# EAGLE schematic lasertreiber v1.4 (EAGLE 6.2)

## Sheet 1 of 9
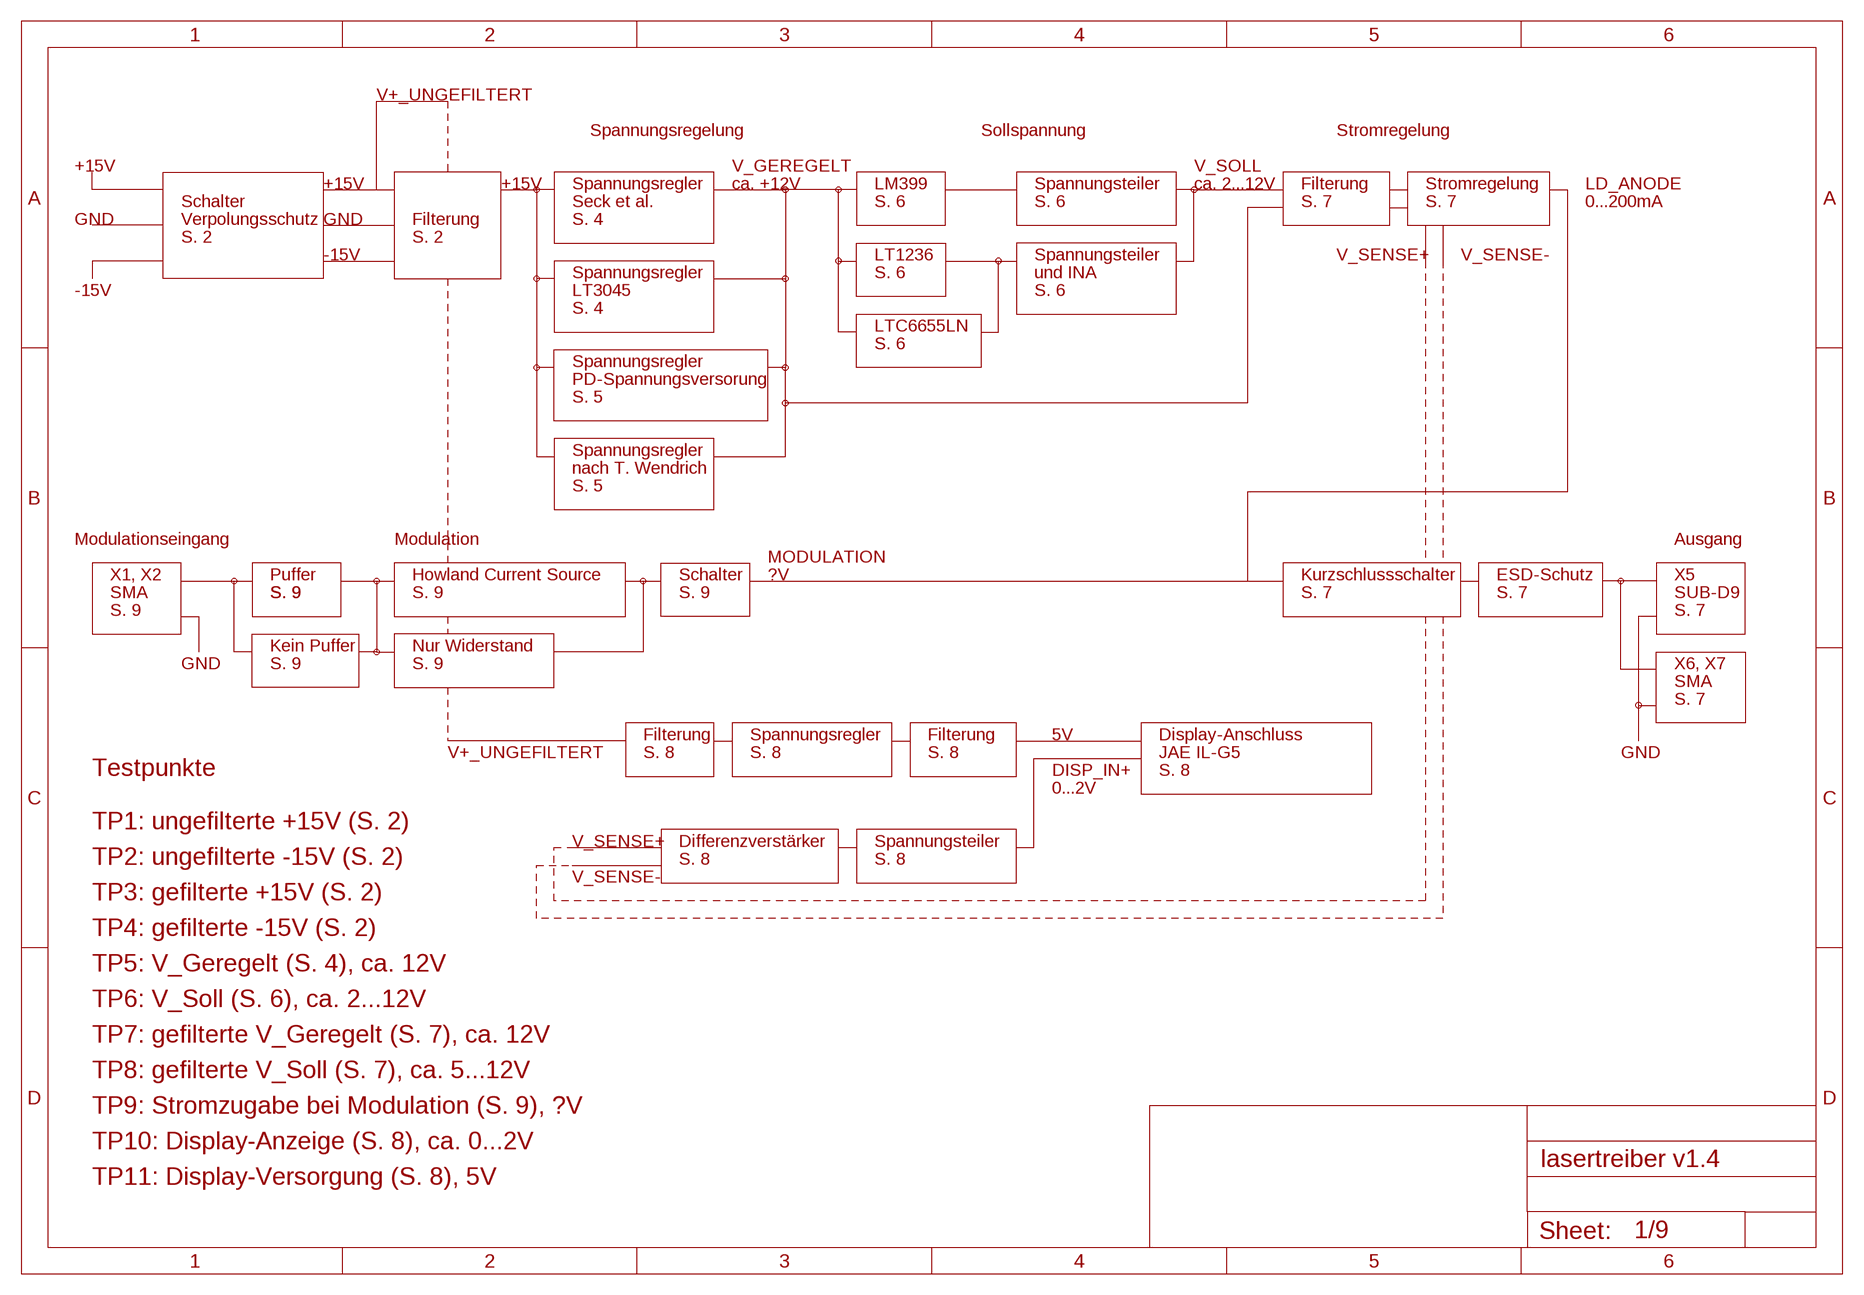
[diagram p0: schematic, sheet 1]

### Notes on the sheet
- V+_UNGEFILTERT
- Spannungsregelung | Sollspannung | Stromregelung
- +15V | V_GEREGELT | V_SOLL
- +15V | +15V | Spannungsregler | ca. +12V | LM399 | Spannungsteiler | ca. 2...12V | Filterung | Stromregelung | LD_ANODE
- Schalter | Seck et al. | S. 6 | S. 6 | S. 7 | S. 7 | 0...200mA
- GND | Verpolungsschutz | GND | Filterung | S. 4
- S. 2 | S. 2
- -15V | LT1236 | Spannungsteiler | V_SENSE+ | V_SENSE-
- Spannungsregler | S. 6 | und INA
- -15V | LT3045 | S. 6
- S. 4
- LTC6655LN
- S. 6
- Spannungsregler
- PD-Spannungsversorung
- S. 5
- Spannungsregler
- nach T. Wendrich
- S. 5
- Modulationseingang | Modulation | Ausgang
- MODULATION
- X1, X2 | Puffer | Howland Current Source | Schalter | ?V | Kurzschlussschalter | ESD-Schutz | X5
- SMA | S. 9 | S. 9 | S. 9 | S. 9 | S. 7 | S. 7 | SUB-D9
- S. 9 | S. 7
- Kein Puffer | Nur Widerstand
- GND | S. 9 | S. 9 | X6, X7
- SMA
- S. 7
- Filterung | Spannungsregler | Filterung | 5V | Display-Anschluss
- V+_UNGEFILTERT | S. 8 | S. 8 | S. 8 | JAE IL-G5 | GND
- Testpunkte | DISP_IN+ | S. 8
- 0...2V
- TP1: ungefilterte +15V (S. 2)
- V_SENSE+ | Differenzverstärker | Spannungsteiler
- TP2: ungefilterte -15V (S. 2) | S. 8 | S. 8
- V_SENSE-
- TP3: gefilterte +15V (S. 2)
- TP4: gefilterte -15V (S. 2)
- TP5: V_Geregelt (S. 4), ca. 12V
- TP6: V_Soll (S. 6), ca. 2...12V
- TP7: gefilterte V_Geregelt (S. 7), ca. 12V
- TP8: gefilterte V_Soll (S. 7), ca. 5...12V
- TP9: Stromzugabe bei Modulation (S. 9), ?V
- TP10: Display-Anzeige (S. 8), ca. 0...2V
- TP11: Display-Versorgung (S. 8), 5V

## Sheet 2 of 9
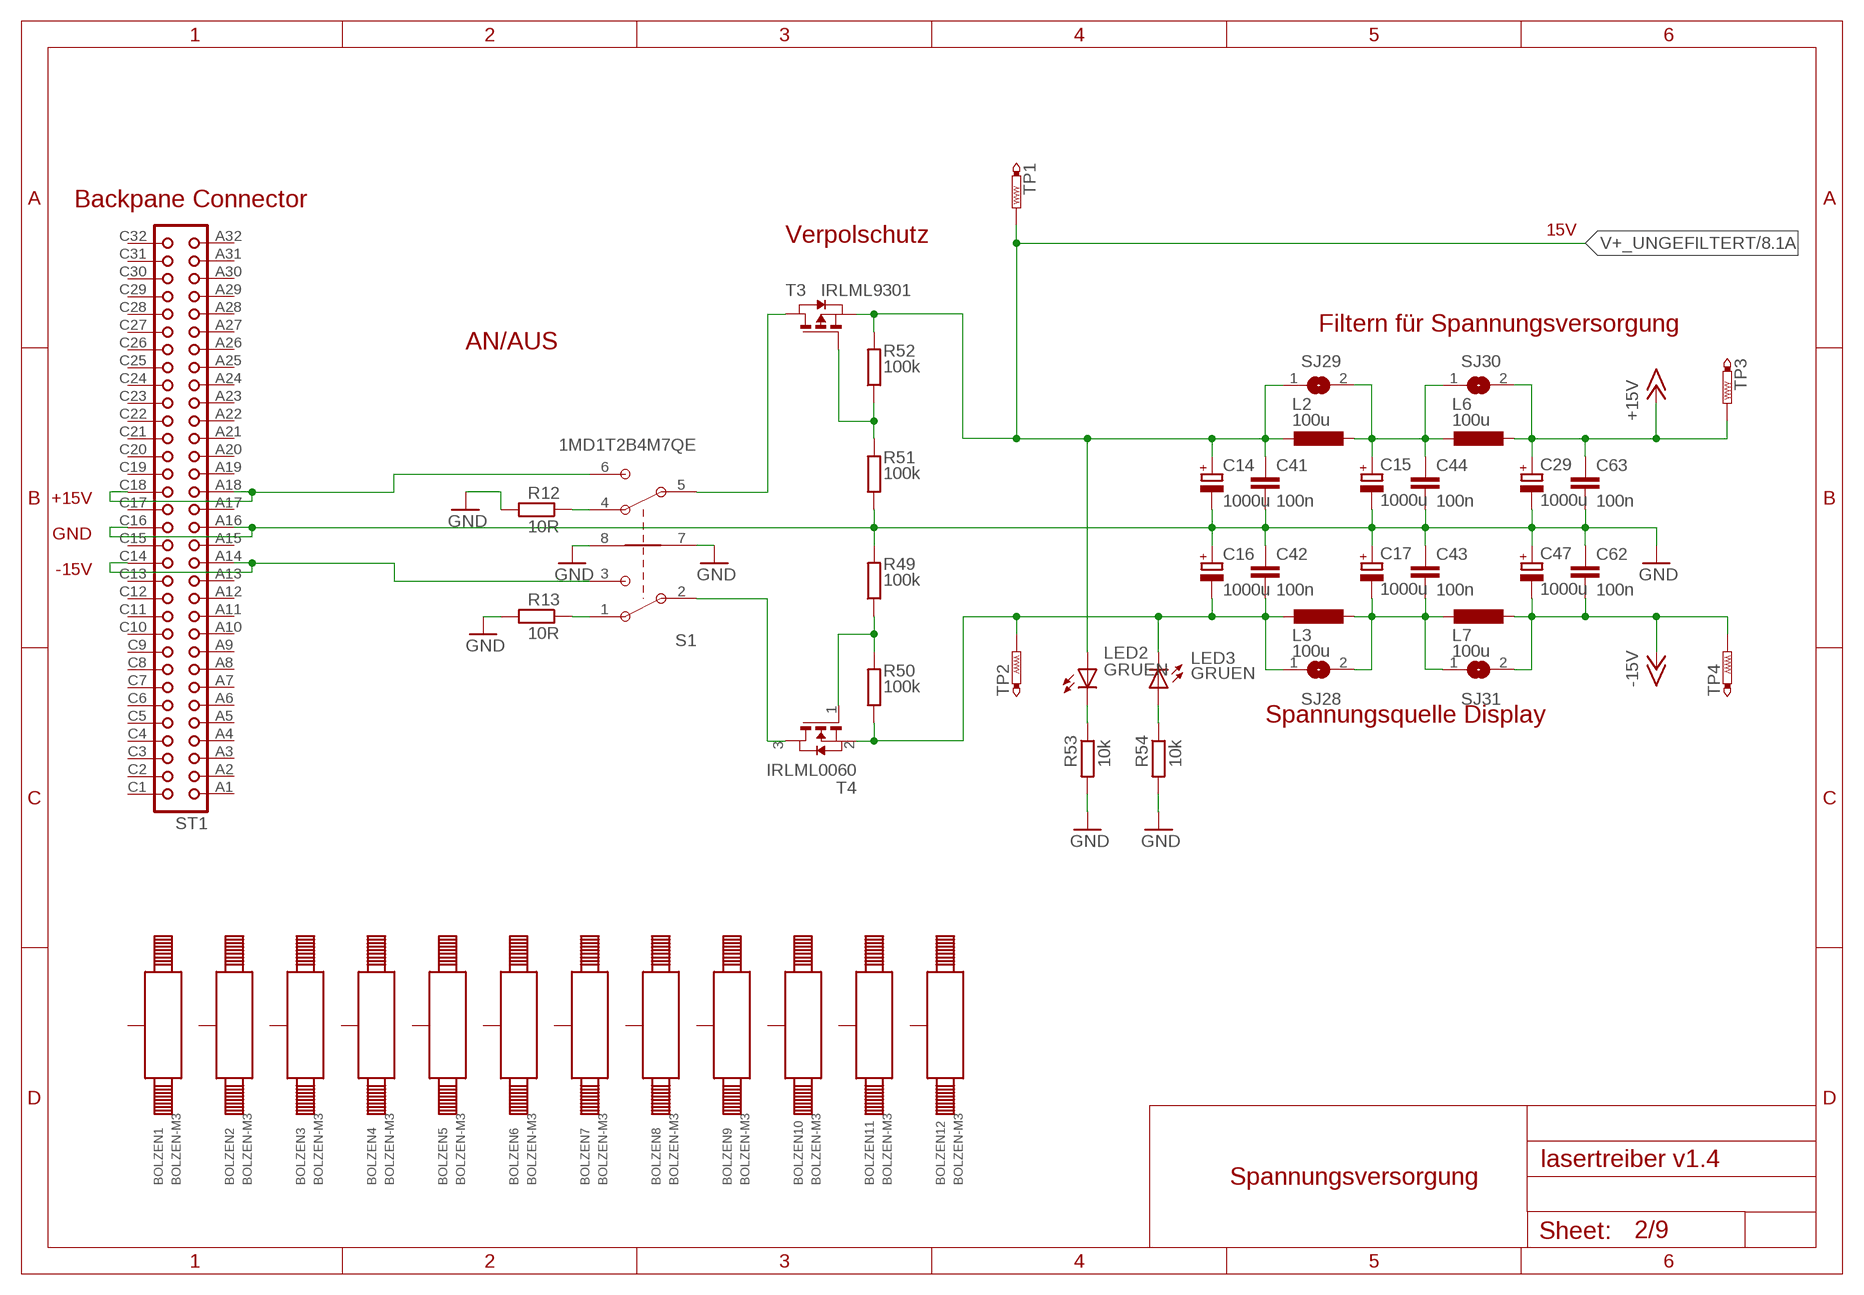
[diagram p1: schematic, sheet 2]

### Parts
BOLZEN1  BOLZEN-M3  [LOCH-M3]
BOLZEN2  BOLZEN-M3  [LOCH-M3]
BOLZEN3  BOLZEN-M3  [LOCH-M3]
BOLZEN4  BOLZEN-M3  [LOCH-M3]
BOLZEN5  BOLZEN-M3  [LOCH-M3]
BOLZEN6  BOLZEN-M3  [LOCH-M3]
BOLZEN7  BOLZEN-M3  [LOCH-M3]
BOLZEN8  BOLZEN-M3  [LOCH-M3]
BOLZEN9  BOLZEN-M3  [LOCH-M3]
BOLZEN10  BOLZEN-M3  [LOCH-M3]
BOLZEN11  BOLZEN-M3  [LOCH-M3]
BOLZEN12  BOLZEN-M3  [LOCH-M3]
C14  1000u  C-POL1000UF  [TT5D10]
C15  1000u  C-POL1000UF  [TT5D10]
C16  1000u  C-POL1000UF  [TT5D10]
C17  1000u  C-POL1000UF  [TT5D10]
C29  1000u  C-POL1000UF  [TT5D10]
C41  100n  C0805  [C0805]
C42  100n  C0805  [C0805]
C43  100n  C0805  [C0805]
C44  100n  C0805  [C0805]
C47  1000u  C-POL1000UF  [TT5D10]
C62  100n  C0805  [C0805]
C63  100n  C0805  [C0805]
L2  100u  L2100MA100UH  [L-GROSS]
L3  100u  L2100MA100UH  [L-GROSS]
L6  100u  L2100MA100UH  [L-GROSS]
L7  100u  L2100MA100UH  [L-GROSS]
LED2  GRUEN  LED3MM-GRUEN  [LED3MM]
LED3  GRUEN  LED3MM-GRUEN  [LED3MM]
R12  10R  R0805  [R0805]
R13  10R  R0805  [R0805]
R49  100k  R0805  [R0805]
R50  100k  R0805  [R0805]
R51  100k  R0805  [R0805]
R52  100k  R0805  [R0805]
R53  10k  R0805  [R0805]
R54  10k  R0805  [R0805]
S1  1MD1T2B4M7QE  [1MD1T2B4M7QE]
SJ28  SJ  [SJ]
SJ29  SJ  [SJ]
SJ30  SJ  [SJ]
SJ31  SJ  [SJ]
ST1  A.KO-09_MAC64LEMESSERLEISTE  [A.KO-09_MAC64L]
T3  IRLML9301  [SOT23]
T4  IRLML0060  [SOT23]
TP1  PTR1PAD1-13  [P1-13]
TP2  PTR1PAD1-13  [P1-13]
TP3  PTR1PAD1-13  [P1-13]
TP4  PTR1PAD1-13  [P1-13]

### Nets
+15V: C29.+ C63.1 L6.P$2 SJ30.2 TP3.TP ; also sheet 3,4,5,6,7,8
-15V: C47.- C62.2 L7.P$2 SJ31.2 TP4.TP ; also sheet 3,6,7,8
GND: C14.- C15.- C16.+ C17.+ C29.- C41.2 C42.1 C43.1 C44.2 C47.+ C62.1 C63.2 R12.2 R13.2 R49.2 R51.1 R53.2 R54.2 S1.7(GND) S1.8(GND) ST1.A16 ST1.C16 ; also sheet 3,4,5,6,7,8,9
N$16: C15.+ C44.1 L2.P$2 L6.P$1 SJ29.2 SJ30.1
N$17: R12.1 S1.4(B1)
N$18: R13.1 S1.1(A1)
N$40: S1.2(A) T4.3(D)
N$54: LED3.A R54.1
N$73: S1.6(B2) ST1.A18 ST1.C18
N$86: R51.2 R52.1 T3.1(G)
N$89: R49.1 R50.2 T4.1(G)
N$97: S1.5(B) T3.3(D)
N$162: S1.3(A2) ST1.A14 ST1.C14
N$175: LED2.K(C) R53.1
V+_UNGEFILTERT: C14.+ C41.1 L2.P$1 LED2.A R52.2 SJ29.1 T3.2(S) TP1.TP ; also sheet 8
V-: C17.- C43.2 L3.P$2 L7.P$1 SJ28.2 SJ31.1
V-_UNGEFILTERT: C16.- C42.2 L3.P$1 LED3.K(C) R50.1 SJ28.1 T4.2(S) TP2.TP
Unconnected: BOLZEN1.1 BOLZEN2.1 BOLZEN3.1 BOLZEN4.1 BOLZEN5.1 BOLZEN6.1 BOLZEN7.1 BOLZEN8.1 BOLZEN9.1 BOLZEN10.1 BOLZEN11.1 BOLZEN12.1 ST1.A1 ST1.A2 ST1.A3 ST1.A4 ST1.A5 ST1.A6 ST1.A7 ST1.A8 ST1.A9 ST1.A10 ST1.A11 ST1.A12 ST1.A13 ST1.A15 ST1.A17 ST1.A19 ST1.A20 ST1.A21 ST1.A22 ST1.A23 ST1.A24 ST1.A25 ST1.A26 ST1.A27 ST1.A28 ST1.A29 ST1.A30 ST1.A31 ST1.A32 ST1.C1 ST1.C2 ST1.C3 ST1.C4 ST1.C5 ST1.C6 ST1.C7 ST1.C8 ST1.C9 ST1.C10 ST1.C11 ST1.C12 ST1.C13 ST1.C15 ST1.C17 ST1.C19 ST1.C20 ST1.C21 ST1.C22 ST1.C23 ST1.C24 ST1.C25 ST1.C26 ST1.C27 ST1.C28 ST1.C29 ST1.C30 ST1.C31 ST1.C32

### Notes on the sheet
- Backpane Connector
- 15V
- Verpolschutz
- Filtern für Spannungsversorgung
- AN/AUS
- +15V
- GND
- -15V
- Spannungsquelle Display
- Spannungsversorgung

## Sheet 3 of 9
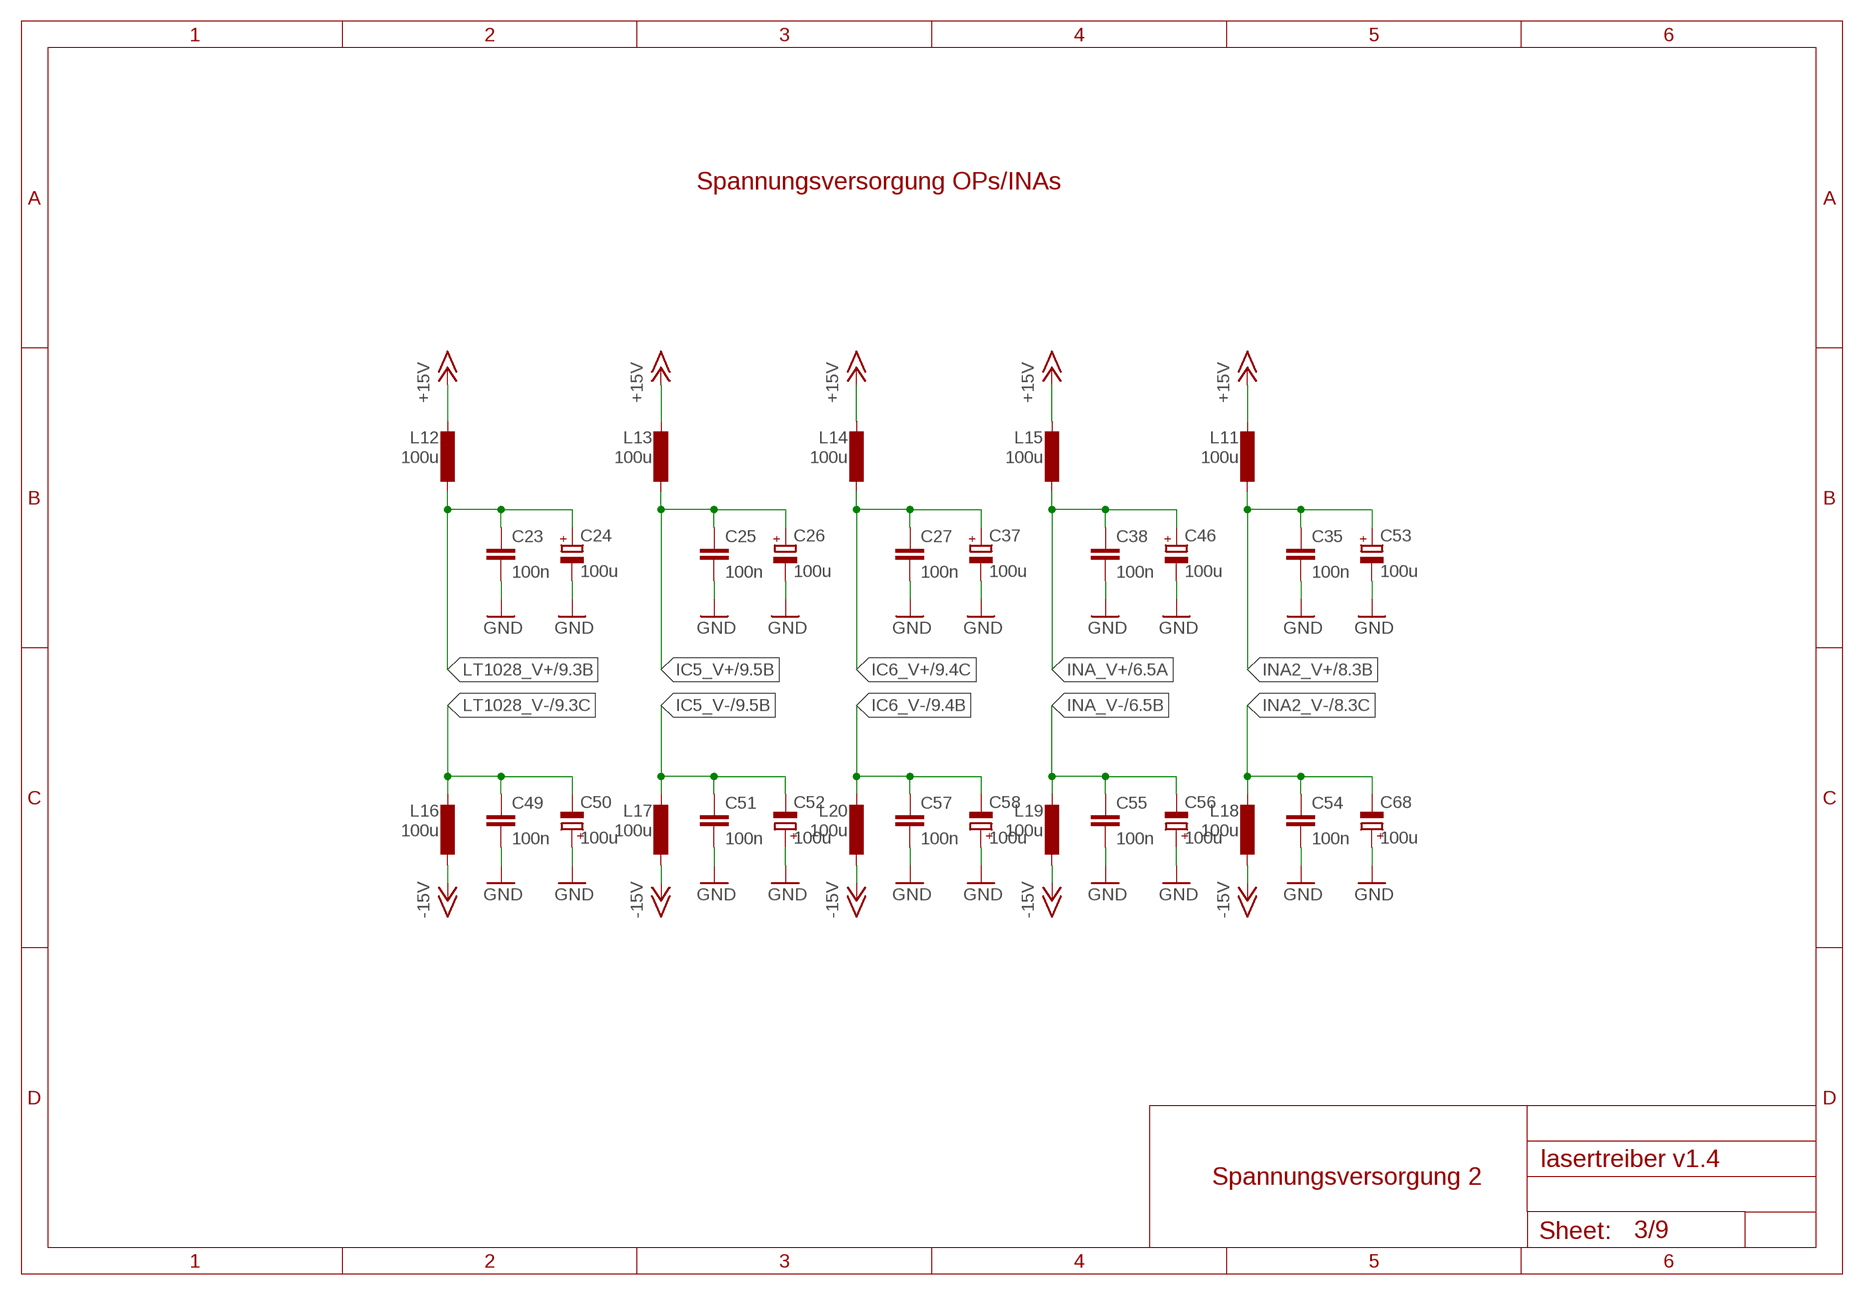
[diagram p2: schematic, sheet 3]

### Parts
C23  100n  C0805  [C0805]
C24  100u  C-POL100UF  [TT5D7]
C25  100n  C0805  [C0805]
C26  100u  C-POL100UF  [TT5D7]
C27  100n  C0805  [C0805]
C35  100n  C0805  [C0805]
C37  100u  C-POL100UF  [TT5D7]
C38  100n  C0805  [C0805]
C46  100u  C-POL100UF  [TT5D7]
C49  100n  C0805  [C0805]
C50  100u  C-POL100UF  [TT5D7]
C51  100n  C0805  [C0805]
C52  100u  C-POL100UF  [TT5D7]
C53  100u  C-POL100UF  [TT5D7]
C54  100n  C0805  [C0805]
C55  100n  C0805  [C0805]
C56  100u  C-POL100UF  [TT5D7]
C57  100n  C0805  [C0805]
C58  100u  C-POL100UF  [TT5D7]
C68  100u  C-POL100UF  [TT5D7]
L11  100u  L100MA100UH  [L-KLEIN]
L12  100u  L100MA100UH  [L-KLEIN]
L13  100u  L100MA100UH  [L-KLEIN]
L14  100u  L100MA100UH  [L-KLEIN]
L15  100u  L100MA100UH  [L-KLEIN]
L16  100u  L100MA100UH  [L-KLEIN]
L17  100u  L100MA100UH  [L-KLEIN]
L18  100u  L100MA100UH  [L-KLEIN]
L19  100u  L100MA100UH  [L-KLEIN]
L20  100u  L100MA100UH  [L-KLEIN]

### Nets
+15V: L11.2 L12.2 L13.2 L14.2 L15.2 ; also sheet 2,4,5,6,7,8
-15V: L16.1 L17.1 L18.1 L19.1 L20.1 ; also sheet 2,6,7,8
GND: C23.2 C24.- C25.2 C26.- C27.2 C35.2 C37.- C38.2 C46.- C49.2 C50.+ C51.2 C52.+ C53.- C54.2 C55.2 C56.+ C57.2 C58.+ C68.+ ; also sheet 2,4,5,6,7,8,9
IC5_V+: C25.1 C26.+ L13.1 ; also sheet 9
IC5_V-: C51.1 C52.- L17.2 ; also sheet 9
IC6_V+: C27.1 C37.+ L14.1 ; also sheet 9
IC6_V-: C57.1 C58.- L20.2 ; also sheet 9
INA2_V+: C35.1 C53.+ L11.1 ; also sheet 8
INA2_V-: C54.1 C68.- L18.2 ; also sheet 8
INA_V+: C38.1 C46.+ L15.1 ; also sheet 6
INA_V-: C55.1 C56.- L19.2 ; also sheet 6
LT1028_V+: C23.1 C24.+ L12.1 ; also sheet 9
LT1028_V-: C49.1 C50.- L16.2 ; also sheet 9

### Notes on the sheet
- Spannungsversorgung OPs/INAs
- Spannungsversorgung 2

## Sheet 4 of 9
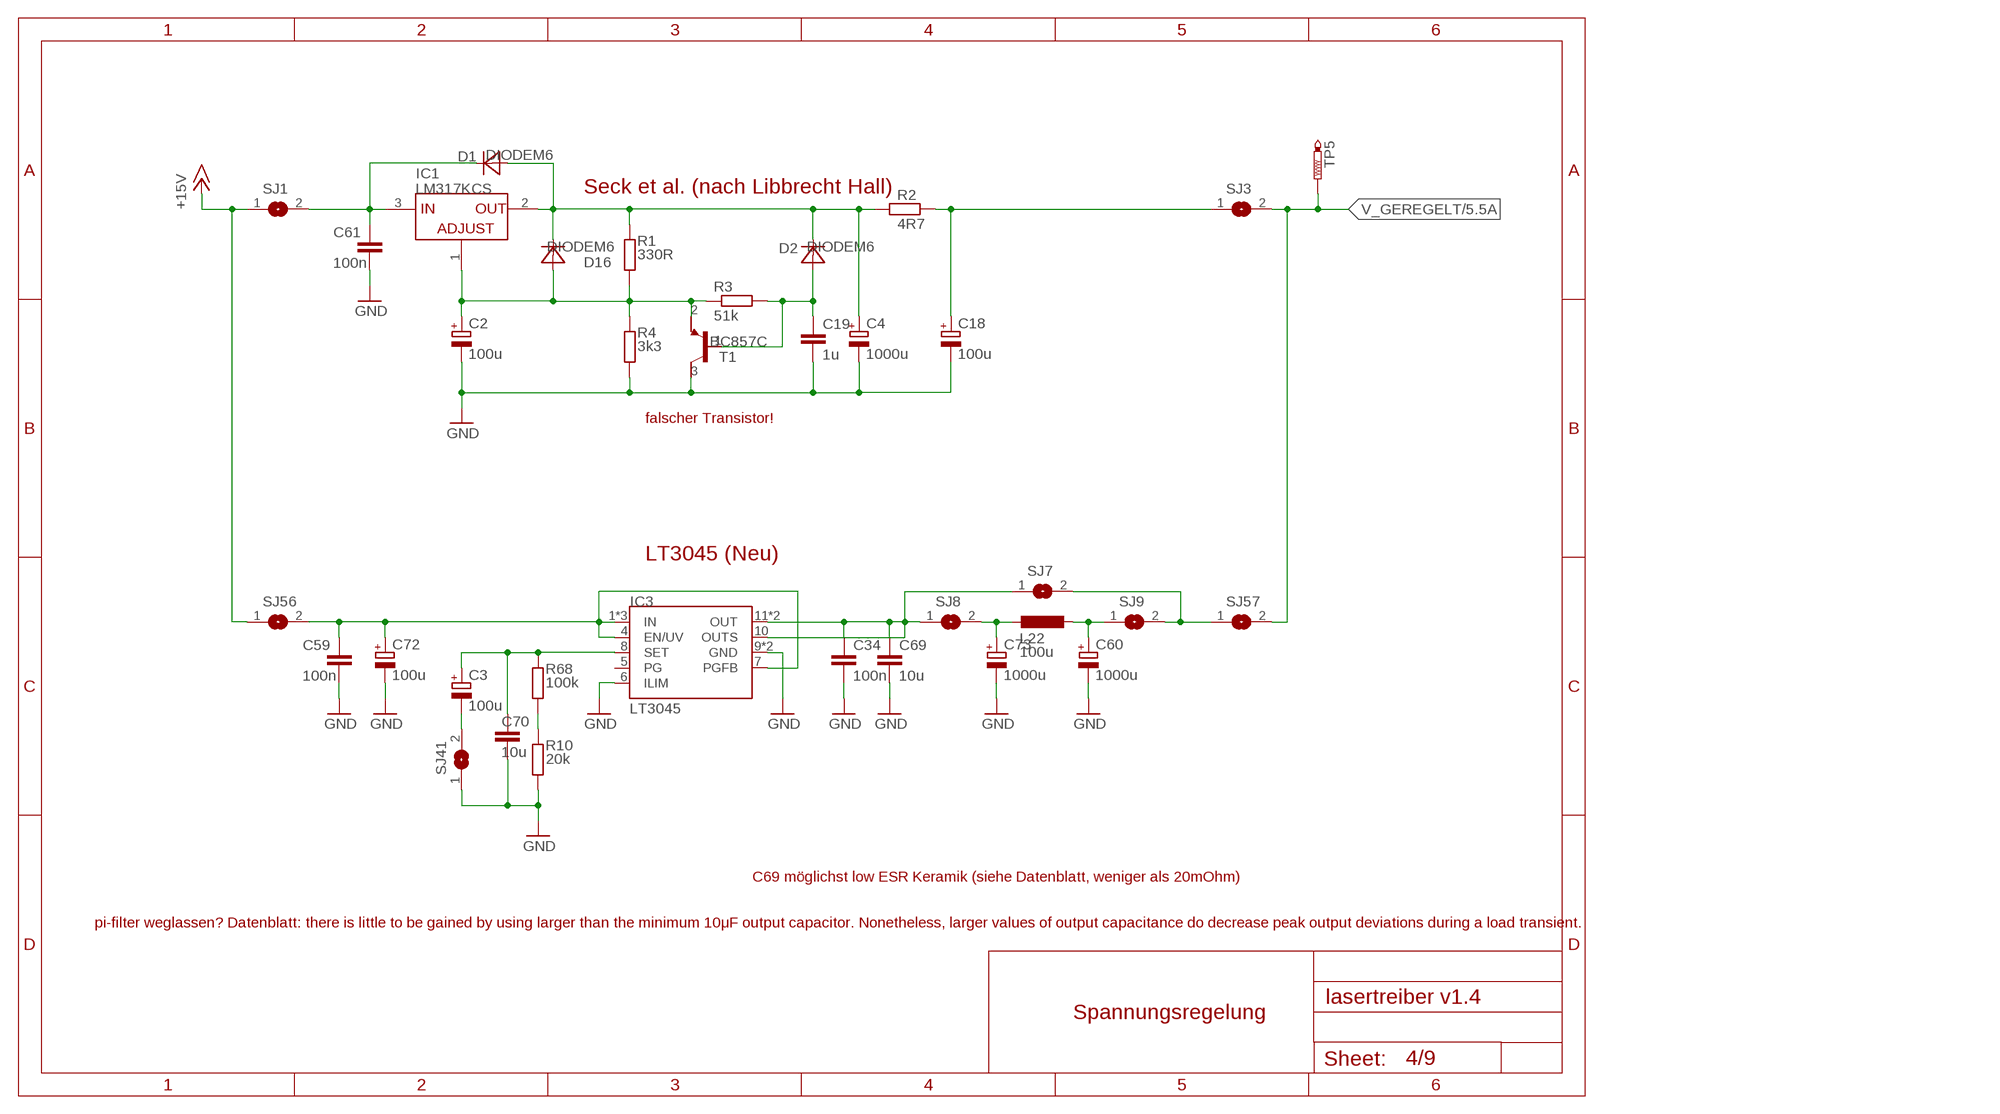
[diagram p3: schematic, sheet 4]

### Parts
C2  100u  C-POL100UF  [TT5D7]
C3  100u  C-POL100UF  [TT5D7]
C4  1000u  C-POL1000UF  [TT5D10]
C18  100u  C-POL100UF  [TT5D7]
C19  1u  C50X75  [C050-050X075]
C34  100n  C0805  [C0805]
C59  100n  C0805  [C0805]
C60  1000u  C-POL1000UF  [TT5D10]
C61  100n  C0805  [C0805]
C69  10u  CMKS2B051001N00KSSD  [MKS2]
C70  10u  CMKS2B051001N00KSSD  [MKS2]
C72  100u  C-POL100UF  [TT5D7]
C73  1000u  C-POL1000UF  [TT5D10]
D1  DIODEM6  [DIODE]
D2  DIODEM6  [DIODE]
D16  DIODEM6  [DIODE]
IC1  LM317KCS  [TO220]
IC3  LT3045  [MSE]
L22  100u  L2100MA100UH  [L-GROSS]
R1  330R  R0805  [R0805]
R2  4R7  R1206  [R1206]
R3  51k  R0805  [R0805]
R4  3k3  R0805  [R0805]
R10  20k  R0805  [R0805]
R68  100k  R0805  [R0805]
SJ1  SJ  [SJ]
SJ3  SJ  [SJ]
SJ7  SJ  [SJ]
SJ8  SJ  [SJ]
SJ9  SJ  [SJ]
SJ41  SJ  [SJ]
SJ56  SJ  [SJ]
SJ57  SJ  [SJ]
T1  BC857C  [SOT23]
TP5  PTR1PAD1-13  [P1-13]

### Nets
+15V: SJ1.1 SJ56.1 ; also sheet 2,3,5,6,7,8
GND: C2.- C4.- C18.- C19.1 C34.1 C59.1 C60.- C61.1 C69.1 C70.1 C72.- C73.- IC3.6(ILIM) IC3.9(GND) IC3.13(GND) R4.1 R10.1 SJ41.1 T1.3(C) ; also sheet 2,3,5,6,7,8,9
N$2: C19.2 D2.ANODE(A) R3.2 T1.1(B)
N$3: C2.+ D16.ANODE(A) IC1.1(ADJUST) R1.1 R3.1 R4.2 T1.2(E)
N$5: C4.+ D1.ANODE(A) D2.KATHODE(C) D16.KATHODE(C) IC1.2(OUT) R1.2 R2.2
N$9: R10.2 R68.1
N$33: C18.+ R2.1 SJ3.1
N$45: C34.2 C69.2 IC3.10(OUTS) IC3.11(OUT) IC3.12(OUT) SJ7.1 SJ8.1
N$46: C73.+ L22.P$1 SJ8.2
N$50: SJ7.2 SJ9.2 SJ57.1
N$51: C3.- SJ41.2
N$138: C3.+ C70.2 IC3.8(SET) R68.2
N$139: C59.2 C72.+ IC3.1(IN) IC3.2(IN) IC3.3(IN) IC3.4(EN/UV) IC3.7(PGFB) SJ56.2
N$142: C60.+ L22.P$2 SJ9.1
V+: C61.2 D1.KATHODE(C) IC1.3(INPUT) SJ1.2
V_GEREGELT: SJ3.2 SJ57.2 TP5.TP ; also sheet 5,6,7
Unconnected: IC3.5(PG)

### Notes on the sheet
- Seck et al. (nach Libbrecht Hall)
- falscher Transistor!
- LT3045 (Neu)
- C69 möglichst low ESR Keramik (siehe Datenblatt, weniger als 20mOhm)
- pi-filter weglassen? Datenblatt: there is little to be gained by using larger than the minimum 10μF output capacitor. Nonetheless, larger values of output capacitance do decrease peak output deviations during a load transient.
- Spannungsregelung

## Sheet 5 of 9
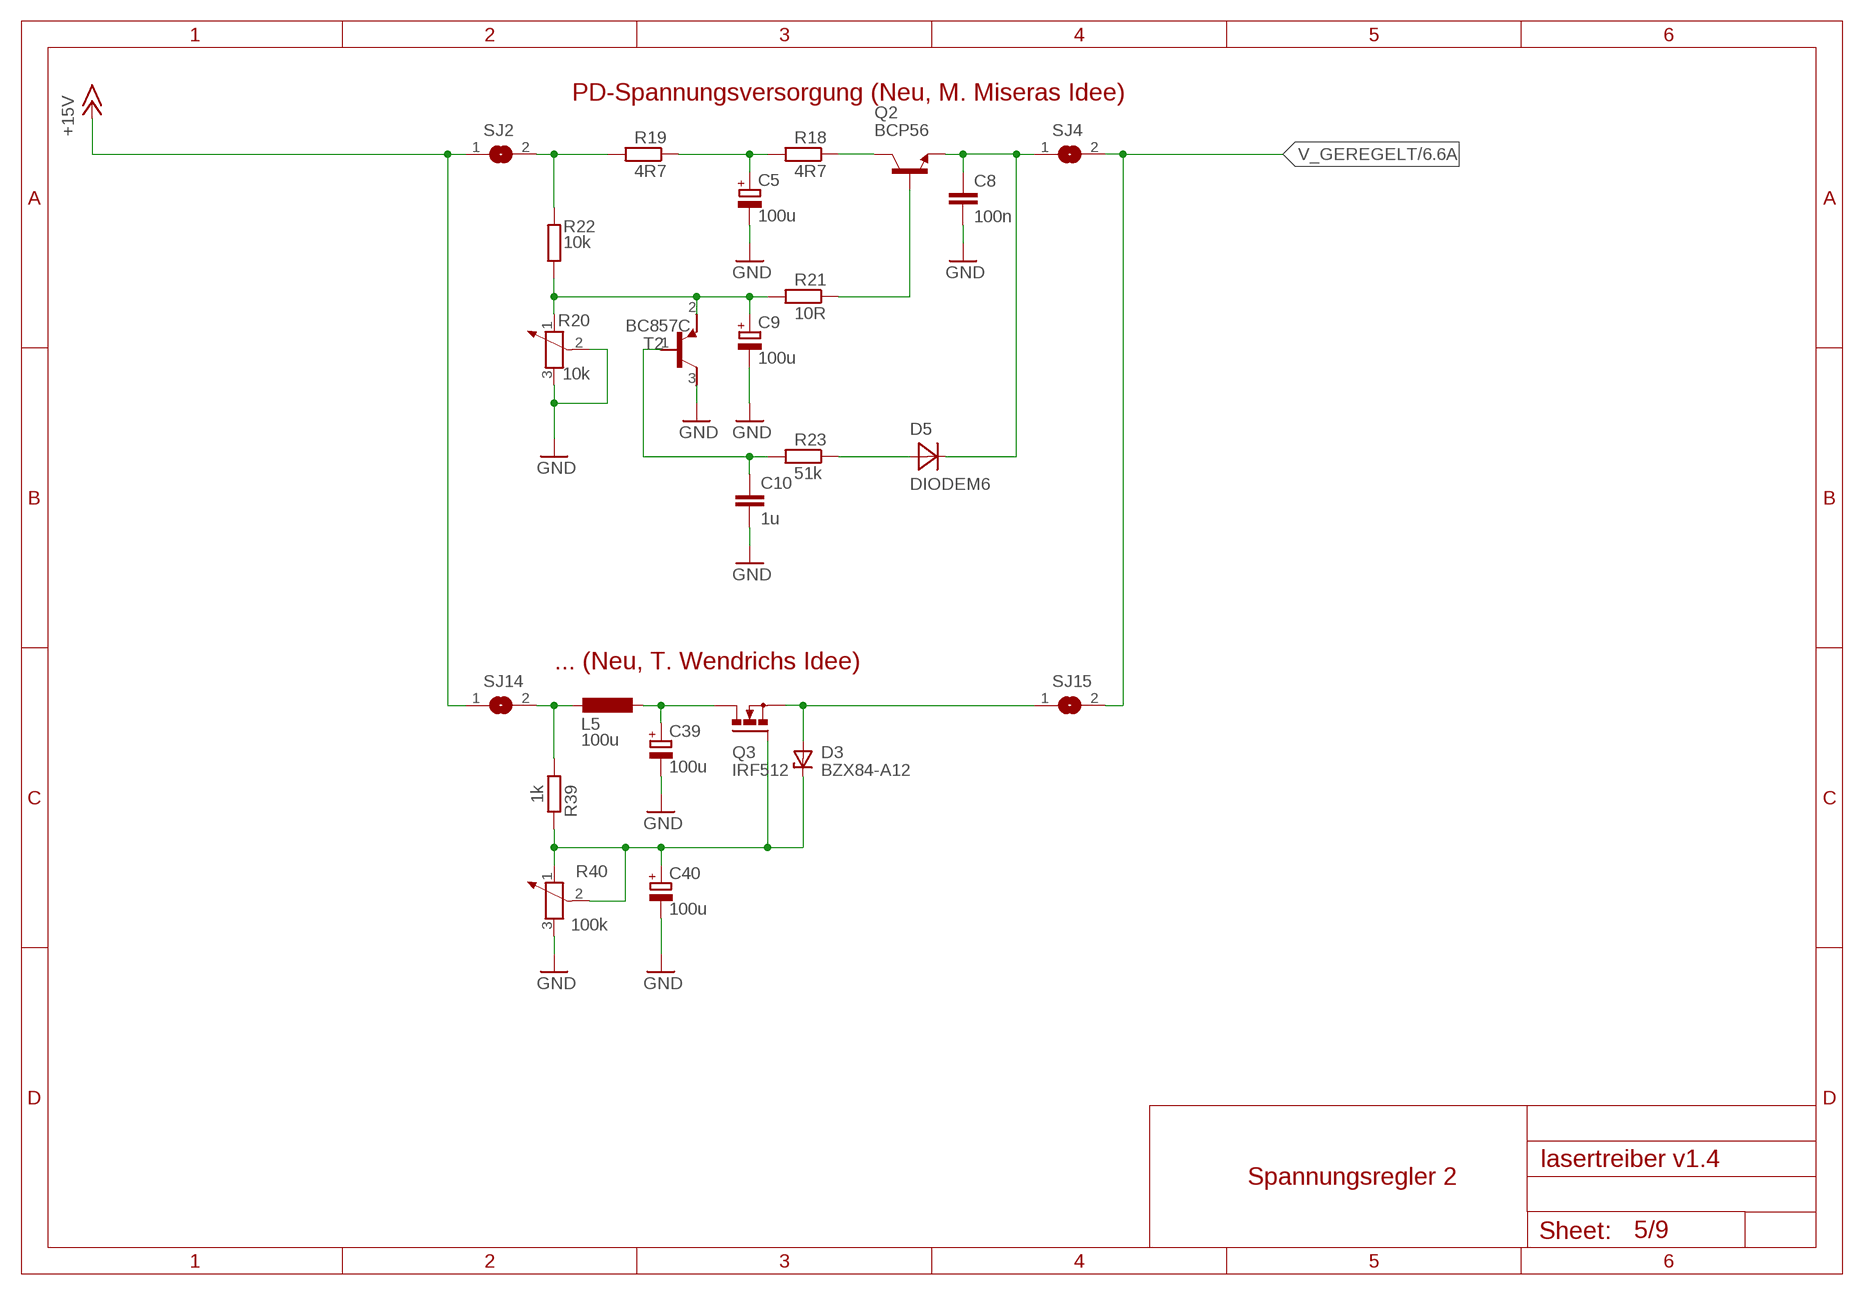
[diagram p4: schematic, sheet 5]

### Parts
C5  100u  C-POL100UF  [TT5D7]
C8  100n  C0805  [C0805]
C9  100u  C-POL100UF  [TT5D7]
C10  1u  C50X75  [C050-050X075]
C39  100u  C-POL100UF  [TT5D7]
C40  100u  C-POL100UF  [TT5D7]
D3  BZX84-A12  BZX84  [SOT23]
D5  DIODEM6  [DIODE]
L5  100u  L2100MA100UH  [L-GROSS]
Q2  BCP56  [SOT223]
Q3  IRF512  [TO220]
R18  4R7  R1206  [R1206]
R19  4R7  R1206  [R1206]
R20  10k  POTENTIOMETER_64Y  [64Y-POTI]
R21  10R  R0805  [R0805]
R22  10k  R0805  [R0805]
R23  51k  R0805  [R0805]
R39  1k  R0805  [R0805]
R40  100k  POTENTIOMETER_64Y  [64Y-POTI]
SJ2  SJ  [SJ]
SJ4  SJ  [SJ]
SJ14  SJ  [SJ]
SJ15  SJ  [SJ]
T2  BC857C  [SOT23]

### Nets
+15V: SJ2.1 SJ14.1 ; also sheet 2,3,4,6,7,8
GND: C5.- C8.1 C9.- C10.1 C39.- C40.- R20.2 R20.3 R40.3 T2.3(C) ; also sheet 2,3,4,6,7,8,9
N$24: C5.+ R18.2 R19.1
N$25: C8.2 D5.KATHODE(C) Q2.3(E) SJ4.1
N$26: Q2.2(C) Q2.4(C) R18.1
N$27: C9.+ R20.1 R21.2 R22.1 T2.2(E)
N$28: Q2.1(B) R21.1
N$29: C10.2 R23.2 T2.1(B)
N$30: R19.2 R22.2 SJ2.2
N$31: D5.ANODE(A) R23.1
N$32: C40.+ D3.3(K) Q3.1(G) R39.1 R40.1 R40.2
N$59: C39.+ L5.P$2 Q3.2(D)
N$60: L5.P$1 R39.2 SJ14.2
N$61: D3.1(A) Q3.3(S) SJ15.1
V_GEREGELT: SJ4.2 SJ15.2 ; also sheet 4,6,7

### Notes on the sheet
- PD-Spannungsversorgung (Neu, M. Miseras Idee)
- ... (Neu, T. Wendrichs Idee)
- Spannungsregler 2

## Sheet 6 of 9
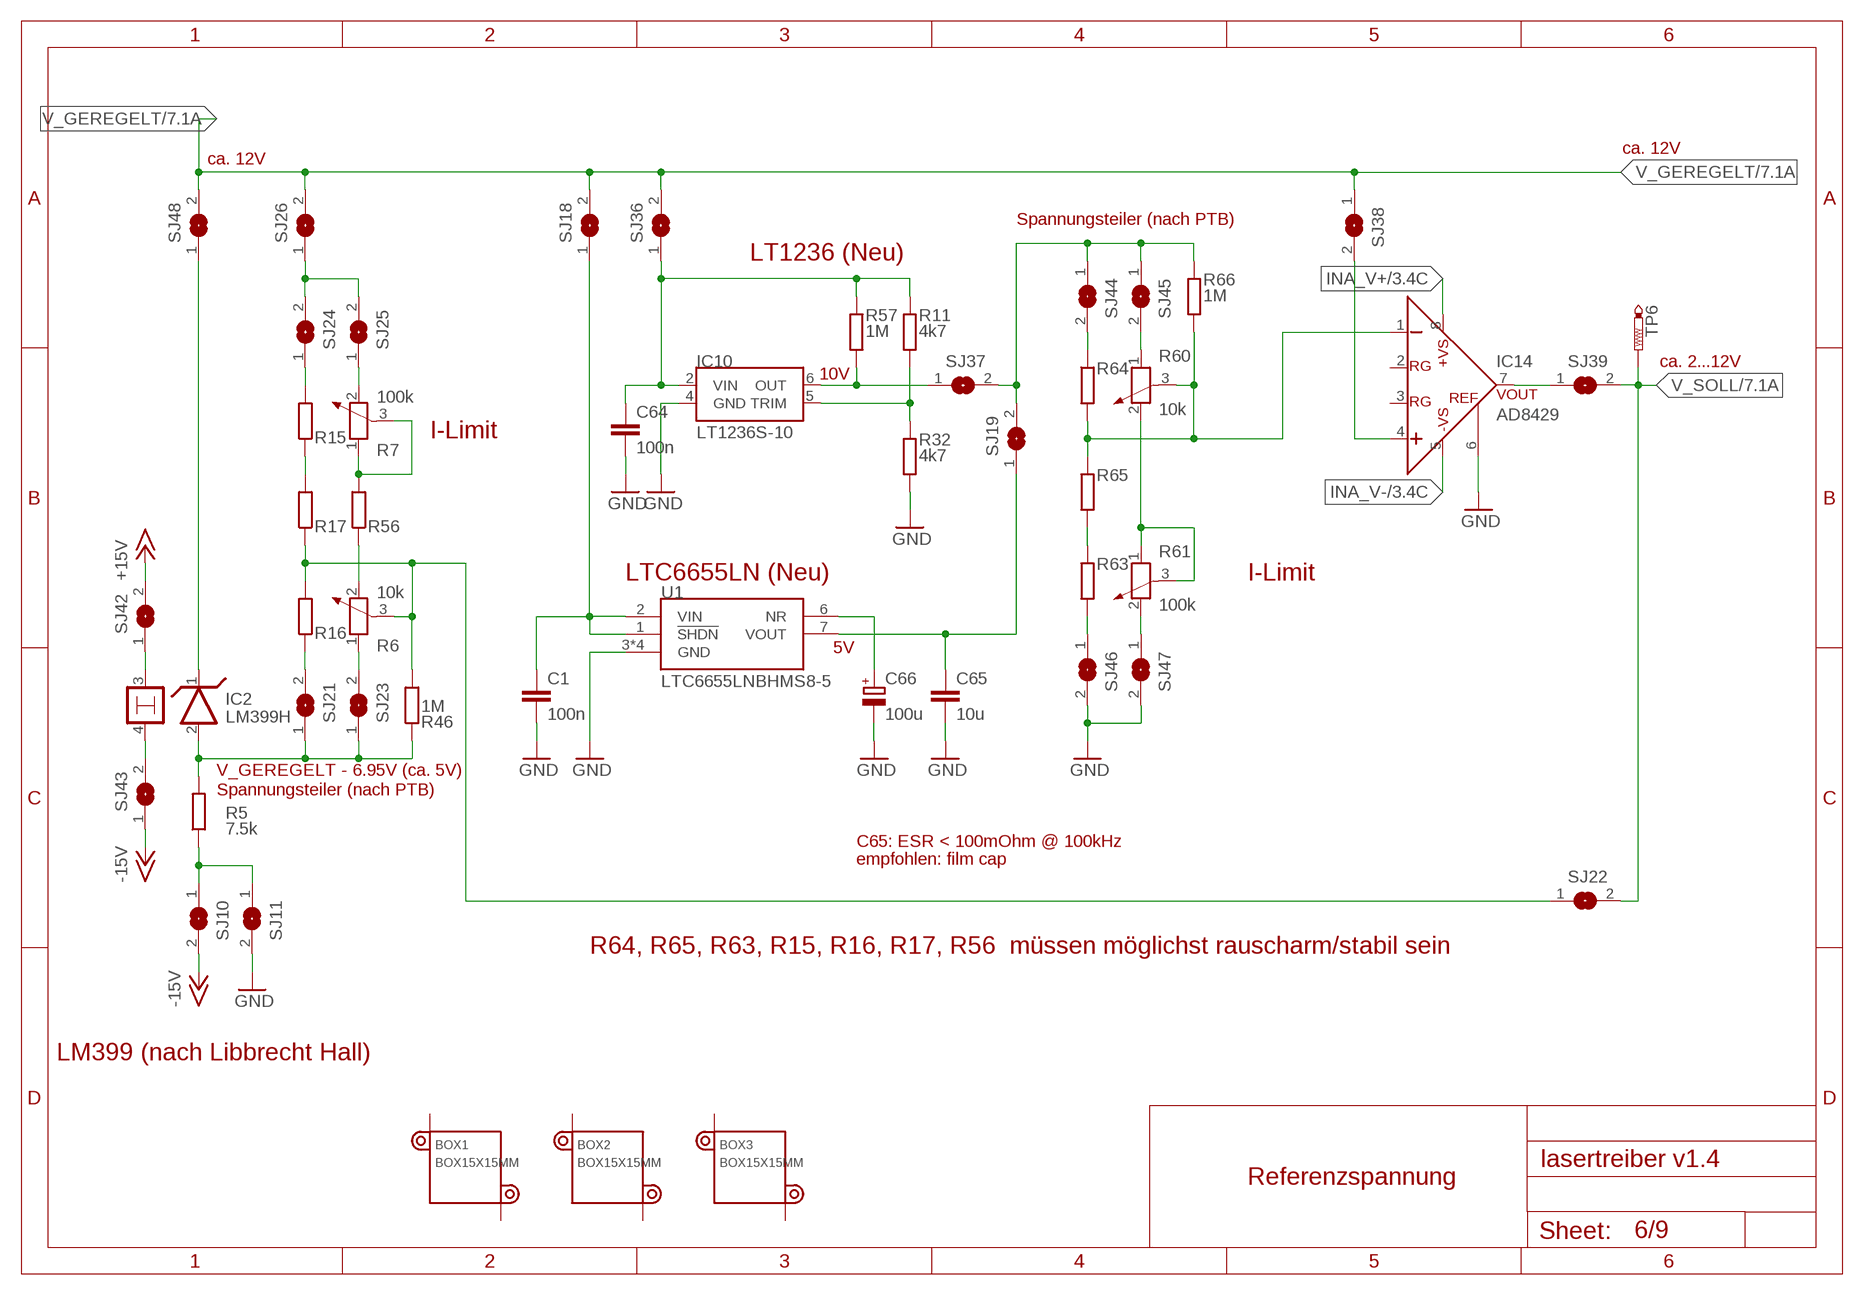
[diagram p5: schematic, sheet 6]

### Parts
BOX1  BOX15X15MM  [BOX-15X15MM]
BOX2  BOX15X15MM  [BOX-15X15MM]
BOX3  BOX15X15MM  [BOX-15X15MM]
C1  100n  C0805  [C0805]
C64  100n  C0805  [C0805]
C65  10u  CMKS2B051001N00KSSD  [MKS2]
C66  100u  C-POL100UF  [TT5D7]
IC2  LM399H  [TO39/4]
IC10  LT1236S-10  [SOIC8]
IC14  AD8429  [R-8]
R5  7.5k  R0805  [R0805]
R6  10k  POTENTIOMETER_PT-10  [PT-10]
R7  100k  POTENTIOMETER_PT-10  [PT-10]
R11  4k7  R0805  [R0805]
R15  R0805  [R0805]
R16  R0805  [R0805]
R17  R0805  [R0805]
R32  4k7  R0805  [R0805]
R46  1M  R0805  [R0805]
R56  R0805  [R0805]
R57  1M  R0805  [R0805]
R60  10k  POTENTIOMETER_PT-10  [PT-10]
R61  100k  POTENTIOMETER_PT-10  [PT-10]
R63  R0805  [R0805]
R64  R0805  [R0805]
R65  R0805  [R0805]
R66  1M  R0805  [R0805]
SJ10  SJ  [SJ]
SJ11  SJ  [SJ]
SJ18  SJ  [SJ]
SJ19  SJ  [SJ]
SJ21  SJ  [SJ]
SJ22  SJ  [SJ]
SJ23  SJ  [SJ]
SJ24  SJ  [SJ]
SJ25  SJ  [SJ]
SJ26  SJ  [SJ]
SJ36  SJ  [SJ]
SJ37  SJ  [SJ]
SJ38  SJ  [SJ]
SJ39  SJ  [SJ]
SJ42  SJ  [SJ]
SJ43  SJ  [SJ]
SJ44  SJ  [SJ]
SJ45  SJ  [SJ]
SJ46  SJ  [SJ]
SJ47  SJ  [SJ]
SJ48  SJ  [SJ]
TP6  PTR1PAD1-13  [P1-13]
U1  LTC6655LNBHMS8-5  [MS8]

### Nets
+15V: SJ42.2 ; also sheet 2,3,4,5,7,8
-15V: SJ10.2 SJ43.1 ; also sheet 2,3,7,8
GND: C1.2 C64.2 C65.2 C66.- IC10.4(GND) IC14.6(REF) R32.2 SJ11.2 SJ46.2 SJ47.2 U1.3(GND) U1.4(GND) U1.5(GND) U1.8(GND) ; also sheet 2,3,4,5,7,8,9
INA_V+: IC14.8(+VIN) ; also sheet 3
INA_V-: IC14.5(-VIN) ; also sheet 3
N$4: IC2.1 SJ48.1
N$7: IC2.2 R5.2 R46.1 SJ21.1 SJ23.1
N$37: SJ24.2 SJ25.2 SJ26.1
N$47: C66.+ U1.6(NR)
N$48: R7.1 R7.3 R56.2
N$57: IC10.5(TRIM) R11.2 R32.1
N$58: IC14.4(+IN) SJ38.2
N$64: R6.1 SJ23.2
N$66: R16.1 SJ21.2
N$71: IC14.7(VOUT) SJ39.1
N$72: R66.1 SJ19.2 SJ37.2 SJ44.1 SJ45.1
N$74: R15.1 R17.2
N$77: R15.2 SJ24.1
N$79: R7.2 SJ25.1
N$83: R6.2 R56.1
N$84: R5.1 SJ10.1 SJ11.1
N$85: R6.3 R16.2 R17.1 R46.2 SJ22.1
N$104: IC10.6(OUT) R57.2 SJ37.1
N$106: C64.1 IC10.2(VIN) R11.1 R57.1 SJ36.1
N$109: IC2.3 SJ42.1
N$117: IC2.4 SJ43.2
N$118: C1.1 SJ18.1 U1.1(!SHDN) U1.2(VIN)
N$119: C65.1 SJ19.1 U1.7(VOUT)
N$121: R60.2 R61.1 R61.3
N$125: R60.1 SJ45.2
N$126: R64.1 SJ44.2
N$127: R63.1 R65.2
N$128: R63.2 SJ46.1
N$129: R61.2 SJ47.1
N$1111: IC14.1(-IN) R60.3 R64.2 R65.1 R66.2
V_GEREGELT: SJ18.2 SJ26.2 SJ36.2 SJ38.1 SJ48.2 ; also sheet 4,5,7
V_SOLL: SJ22.2 SJ39.2 TP6.TP ; also sheet 7
Unconnected: BOX1.1 BOX1.2 BOX2.1 BOX2.2 BOX3.1 BOX3.2 IC14.2(RG) IC14.3(RG)

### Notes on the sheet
- ca. 12V
- ca. 12V
- Spannungsteiler (nach PTB)
- LT1236 (Neu)
- ca. 2...12V
- 10V
- I-Limit
- LTC6655LN (Neu) | I-Limit
- 5V
- V_GEREGELT - 6.95V (ca. 5V)
- Spannungsteiler (nach PTB)
- C65: ESR < 100mOhm @ 100kHz
- empfohlen: film cap
- R64, R65, R63, R15, R16, R17, R56  müssen möglichst rauscharm/stabil sein
- LM399 (nach Libbrecht Hall)
- Referenzspannung

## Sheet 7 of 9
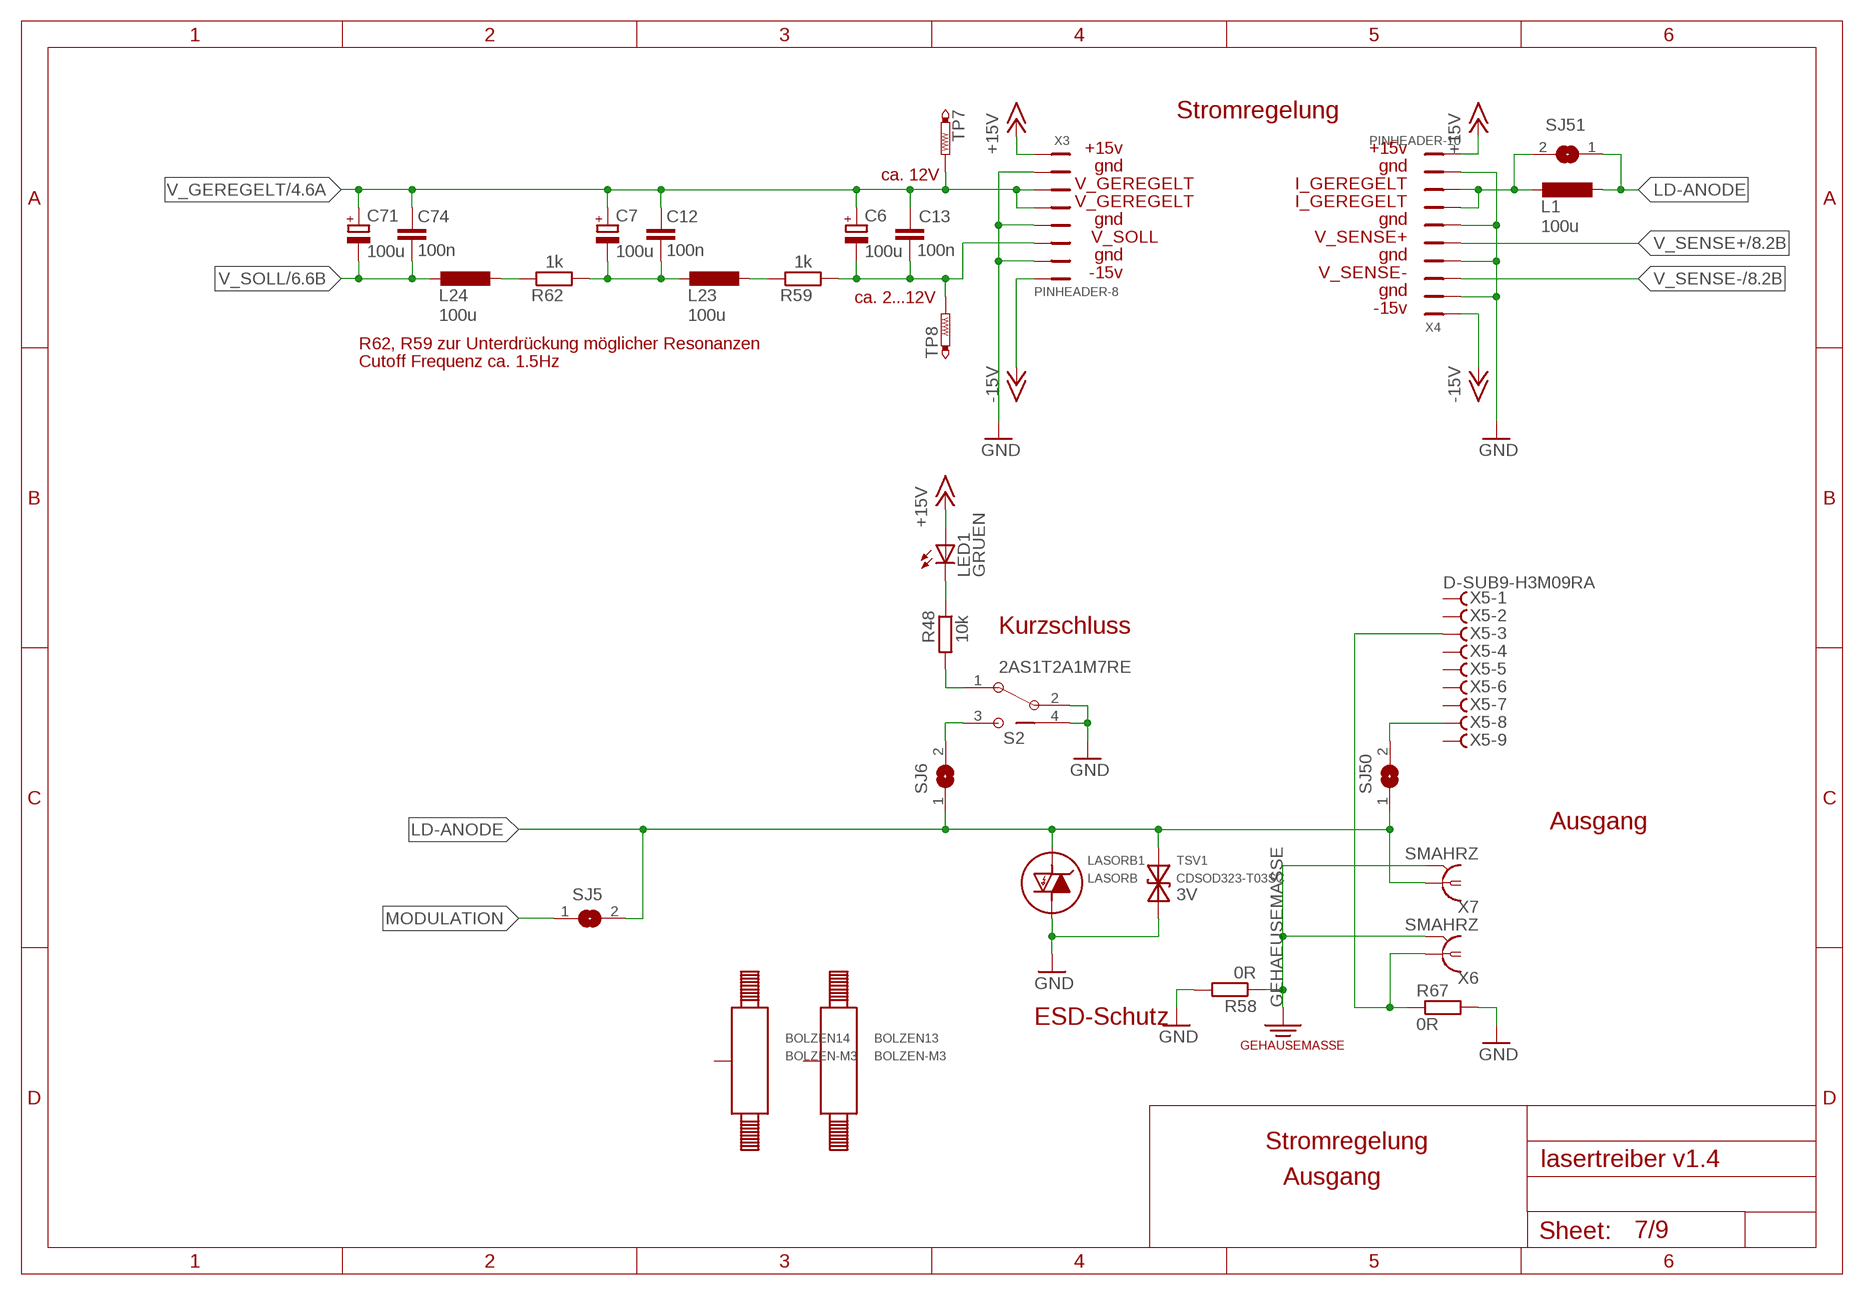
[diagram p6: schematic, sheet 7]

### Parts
BOLZEN13  BOLZEN-M3  [LOCH-M3]
BOLZEN14  BOLZEN-M3  [LOCH-M3]
C6  100u  C-POL100UF  [TT5D7]
C7  100u  C-POL100UF  [TT5D7]
C12  100n  C0805  [C0805]
C13  100n  C0805  [C0805]
C71  100u  C-POL100UF  [TT5D7]
C74  100n  C0805  [C0805]
GEHAEUSE1  GEHAEUSEMASSE  [GEHAEUSEMASSE]
L1  100u  L2100MA100UH  [L-GROSS]
L23  100u  L100MA100UH  [L-KLEIN]
L24  100u  L100MA100UH  [L-KLEIN]
LASORB1  LASORB  [LASORB]
LED1  GRUEN  LED3MM-GRUEN  [LED3MM]
R48  10k  R0805  [R0805]
R58  0R  R0805  [R0805]
R59  1k  R0805  [R0805]
R62  1k  R0805  [R0805]
R67  0R  R0805  [R0805]
S2  2AS1T2A1M7RE  [2AS1T2A1M7RE]
SJ5  SJ  [SJ]
SJ6  SJ  [SJ]
SJ50  SJ  [SJ]
SJ51  SJ  [SJ]
TP7  PTR1PAD1-13  [P1-13]
TP8  PTR1PAD1-13  [P1-13]
TSV1  CDSOD323-T03SC  CDSOD323-TXXSC''  [SOD323-W]
X3  PINHEADER-8  [PINHEADER-8]
X4  PINHEADER-10  [PINHEADER-10]
X5  D-SUB9-H3M09RA  [H3M09RA]
X6  SMAHRZ  [SMA20_HRZ]
X7  SMAHRZ  [SMA20_HRZ]

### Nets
+15V: LED1.A X3.1 X4.10 ; also sheet 2,3,4,5,6,8
-15V: X3.8 X4.1 ; also sheet 2,3,6,8
GEHAEUSEMASSE: GEHAEUSE1.P$2 R58.1 X6.GND@1 X6.GND@2 X6.GND@3 X6.GND@4 X7.GND@1 X7.GND@2 X7.GND@3 X7.GND@4 ; also sheet 9
GND: LASORB1.LDK R58.2 R67.2 S2.2(A) S2.4(GND) TSV1.C X3.2 X3.5 X3.7 X4.2 X4.4 X4.6 X4.9 ; also sheet 2,3,4,5,6,8,9
LD-ANODE: L1.P$2 LASORB1.LDA SJ5.2 SJ6.1 SJ50.1 SJ51.1 TSV1.A X7.SIGNAL
MODULATION: SJ5.1 ; also sheet 9
N$1: C6.- C13.1 R59.2 TP8.TP X3.6
N$8: C7.- C12.1 L23.1 R62.2
N$44: S2.3(A2) SJ6.2
N$49: L1.P$1 SJ51.2 X4.7 X4.8
N$88: L24.2 R62.1
N$90: L23.2 R59.1
N$108: R67.1 X5.3 X6.SIGNAL
N$130: SJ50.2 X5.8
N$173: LED1.K(C) R48.1
N$174: R48.2 S2.1(A1)
V_GEREGELT: C6.+ C7.+ C12.2 C13.2 C71.+ C74.2 TP7.TP X3.3 X3.4 ; also sheet 4,5,6
V_SENSE+: X4.5 ; also sheet 8
V_SENSE-: X4.3 ; also sheet 8
V_SOLL: C71.- C74.1 L24.1 ; also sheet 6
Unconnected: BOLZEN13.1 BOLZEN14.1 X5.1 X5.2 X5.4 X5.5 X5.6 X5.7 X5.9

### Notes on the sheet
- Stromregelung
- +15v | +15v
- gnd | gnd
- ca. 12V
- V_GEREGELT | I_GEREGELT
- V_GEREGELT | I_GEREGELT
- gnd | gnd
- V_SOLL | V_SENSE+
- gnd | gnd
- -15v | V_SENSE-
- gnd
- ca. 2...12V
- -15v
- R62, R59 zur Unterdrückung möglicher Resonanzen
- Cutoff Frequenz ca. 1.5Hz
- Kurzschluss
- Ausgang
- 3V
- ESD-Schutz
- Stromregelung
- Ausgang

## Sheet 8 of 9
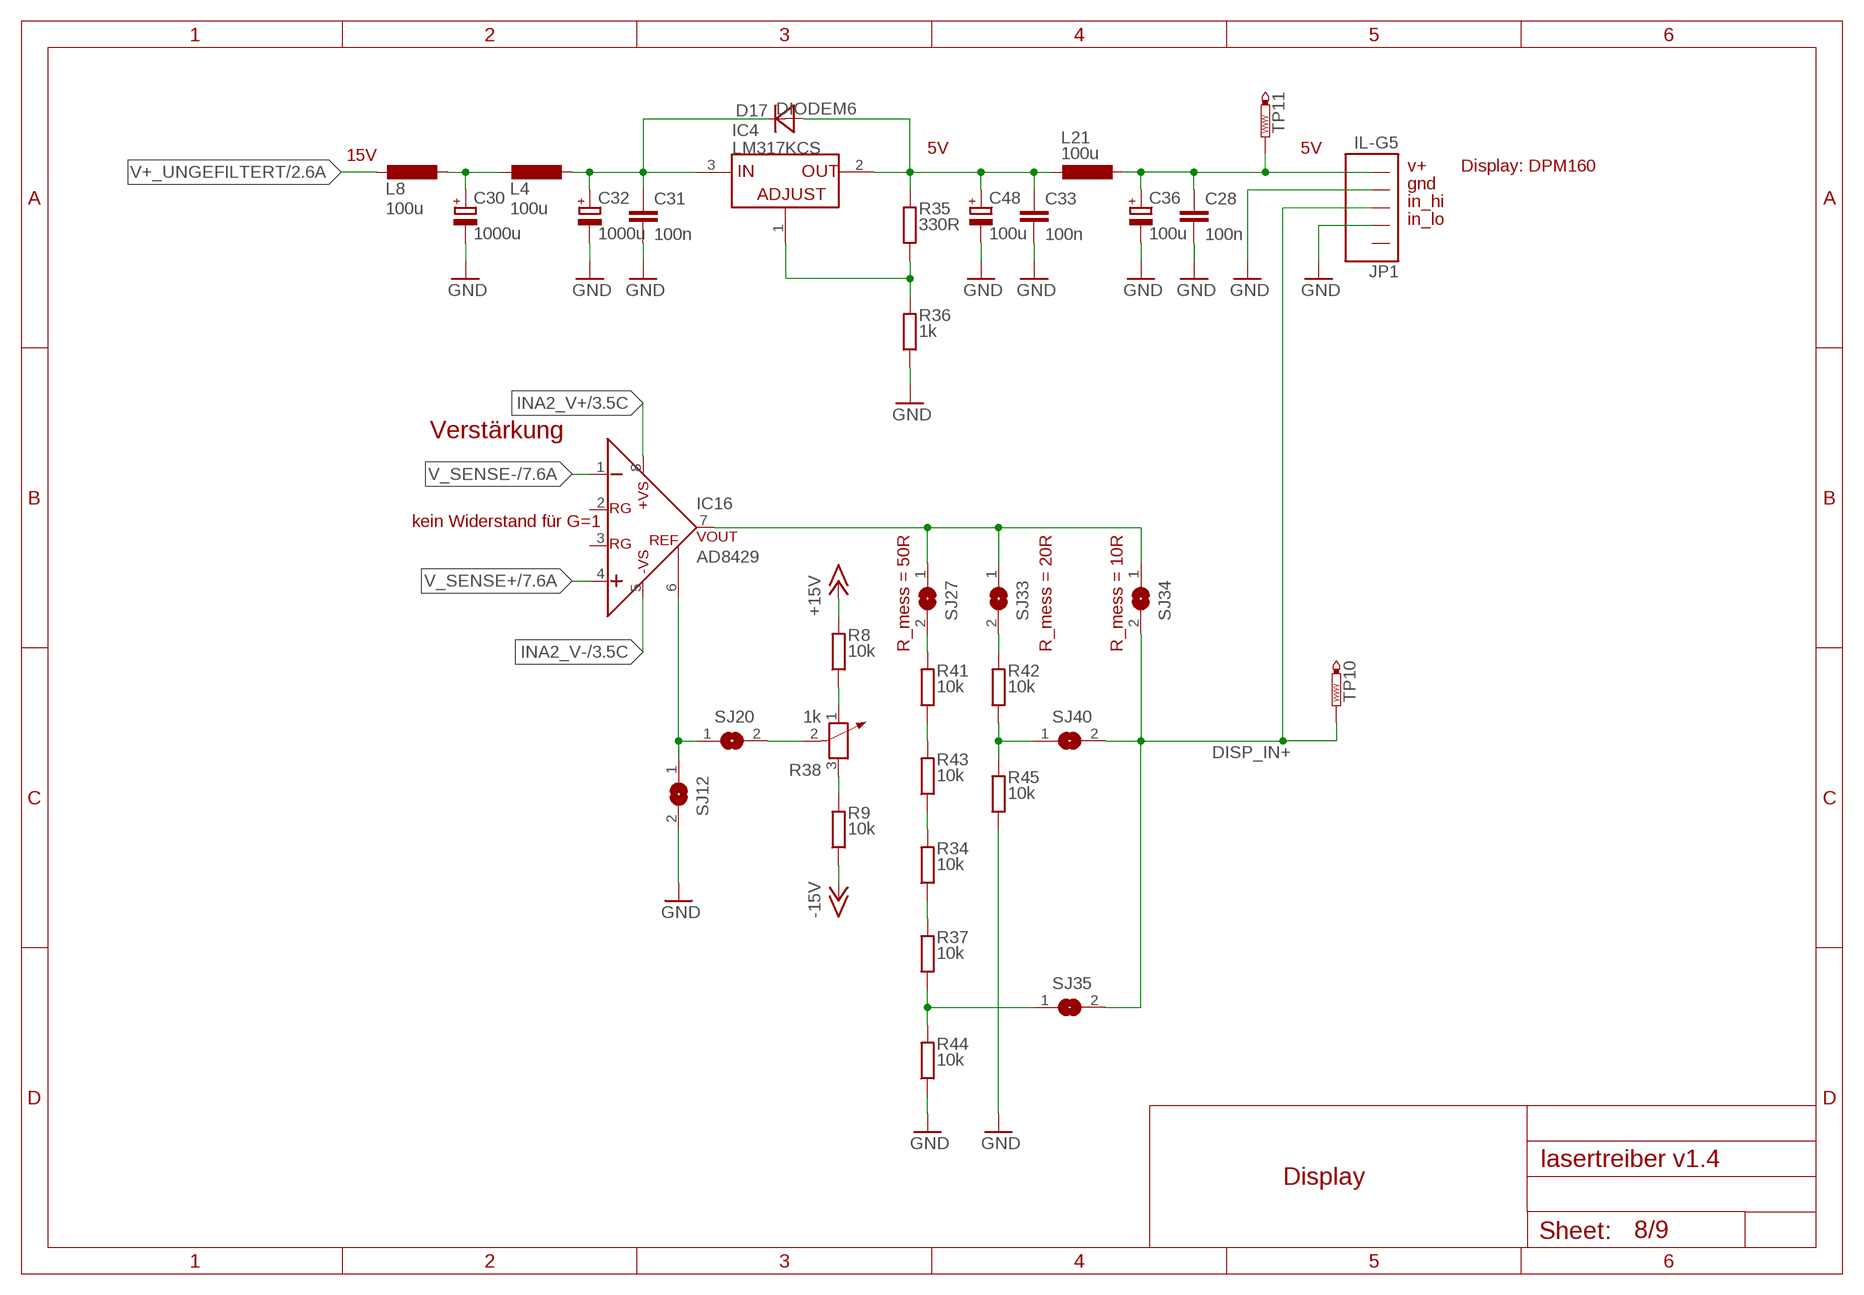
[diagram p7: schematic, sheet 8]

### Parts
C28  100n  C0805  [C0805]
C30  1000u  C-POL1000UF  [TT5D10]
C31  100n  C0805  [C0805]
C32  1000u  C-POL1000UF  [TT5D10]
C33  100n  C0805  [C0805]
C36  100u  C-POL100UF  [TT5D7]
C48  100u  C-POL100UF  [TT5D7]
D17  DIODEM6  [DIODE]
IC4  LM317KCS  [TO220]
IC16  AD8429  [R-8]
JP1  IL-G5  [IL-G5]
L4  100u  L100MA100UH  [L-KLEIN]
L8  100u  L100MA100UH  [L-KLEIN]
L21  100u  L100MA100UH  [L-KLEIN]
R8  10k  R0805  [R0805]
R9  10k  R0805  [R0805]
R34  10k  R0805  [R0805]
R35  330R  R0805  [R0805]
R36  1k  R0805  [R0805]
R37  10k  R0805  [R0805]
R38  1k  POTENTIOMETER_64Y  [64Y-POTI]
R41  10k  R0805  [R0805]
R42  10k  R0805  [R0805]
R43  10k  R0805  [R0805]
R44  10k  R0805  [R0805]
R45  10k  R0805  [R0805]
SJ12  SJ  [SJ]
SJ20  SJ  [SJ]
SJ27  SJ  [SJ]
SJ33  SJ  [SJ]
SJ34  SJ  [SJ]
SJ35  SJ  [SJ]
SJ40  SJ  [SJ]
TP10  PTR1PAD1-13  [P1-13]
TP11  PTR1PAD1-13  [P1-13]

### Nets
+15V: R8.2 ; also sheet 2,3,4,5,6,7
-15V: R9.1 ; also sheet 2,3,6,7
DISP_IN+: JP1.P$3 SJ34.2 SJ35.2 SJ40.2 TP10.TP
DISP_V+: C33.1 C48.+ D17.ANODE(A) IC4.2(OUT) L21.1 R35.2
GND: C28.2 C30.- C31.2 C32.- C33.2 C36.- C48.- JP1.P$2 JP1.P$4 R36.1 R44.1 R45.1 SJ12.2 ; also sheet 2,3,4,5,6,7,9
INA2_V+: IC16.8(+VIN) ; also sheet 3
INA2_V-: IC16.5(-VIN) ; also sheet 3
N$6: R37.1 R44.2 SJ35.1
N$10: R8.1 R38.1
N$11: R34.1 R37.2
N$12: R9.2 R38.3
N$14: IC16.6(REF) SJ12.1 SJ20.1
N$15: R34.2 R43.1
N$19: R38.2 SJ20.2
N$22: IC16.7(VOUT) SJ27.1 SJ33.1 SJ34.1
N$53: R41.2 SJ27.2
N$55: C28.1 C36.+ JP1.P$5 L21.2 TP11.TP
N$56: IC4.1(ADJUST) R35.1 R36.2
N$62: R42.2 SJ33.2
N$63: R42.1 R45.2 SJ40.1
N$69: R41.1 R43.2
N$81: C30.+ L4.1 L8.2
N$135: C31.1 C32.+ D17.KATHODE(C) IC4.3(INPUT) L4.2
V+_UNGEFILTERT: L8.1 ; also sheet 2
V_SENSE+: IC16.4(+IN) ; also sheet 7
V_SENSE-: IC16.1(-IN) ; also sheet 7
Unconnected: IC16.2(RG) IC16.3(RG) JP1.P$1

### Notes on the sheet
- 5V | 5V
- 15V
- v+ | Display: DPM160
- gnd
- in_hi
- in_lo
- Verstärkung
- kein Widerstand für G=1
- R_mess = 50R | R_mess = 20R | R_mess = 10R
- Display

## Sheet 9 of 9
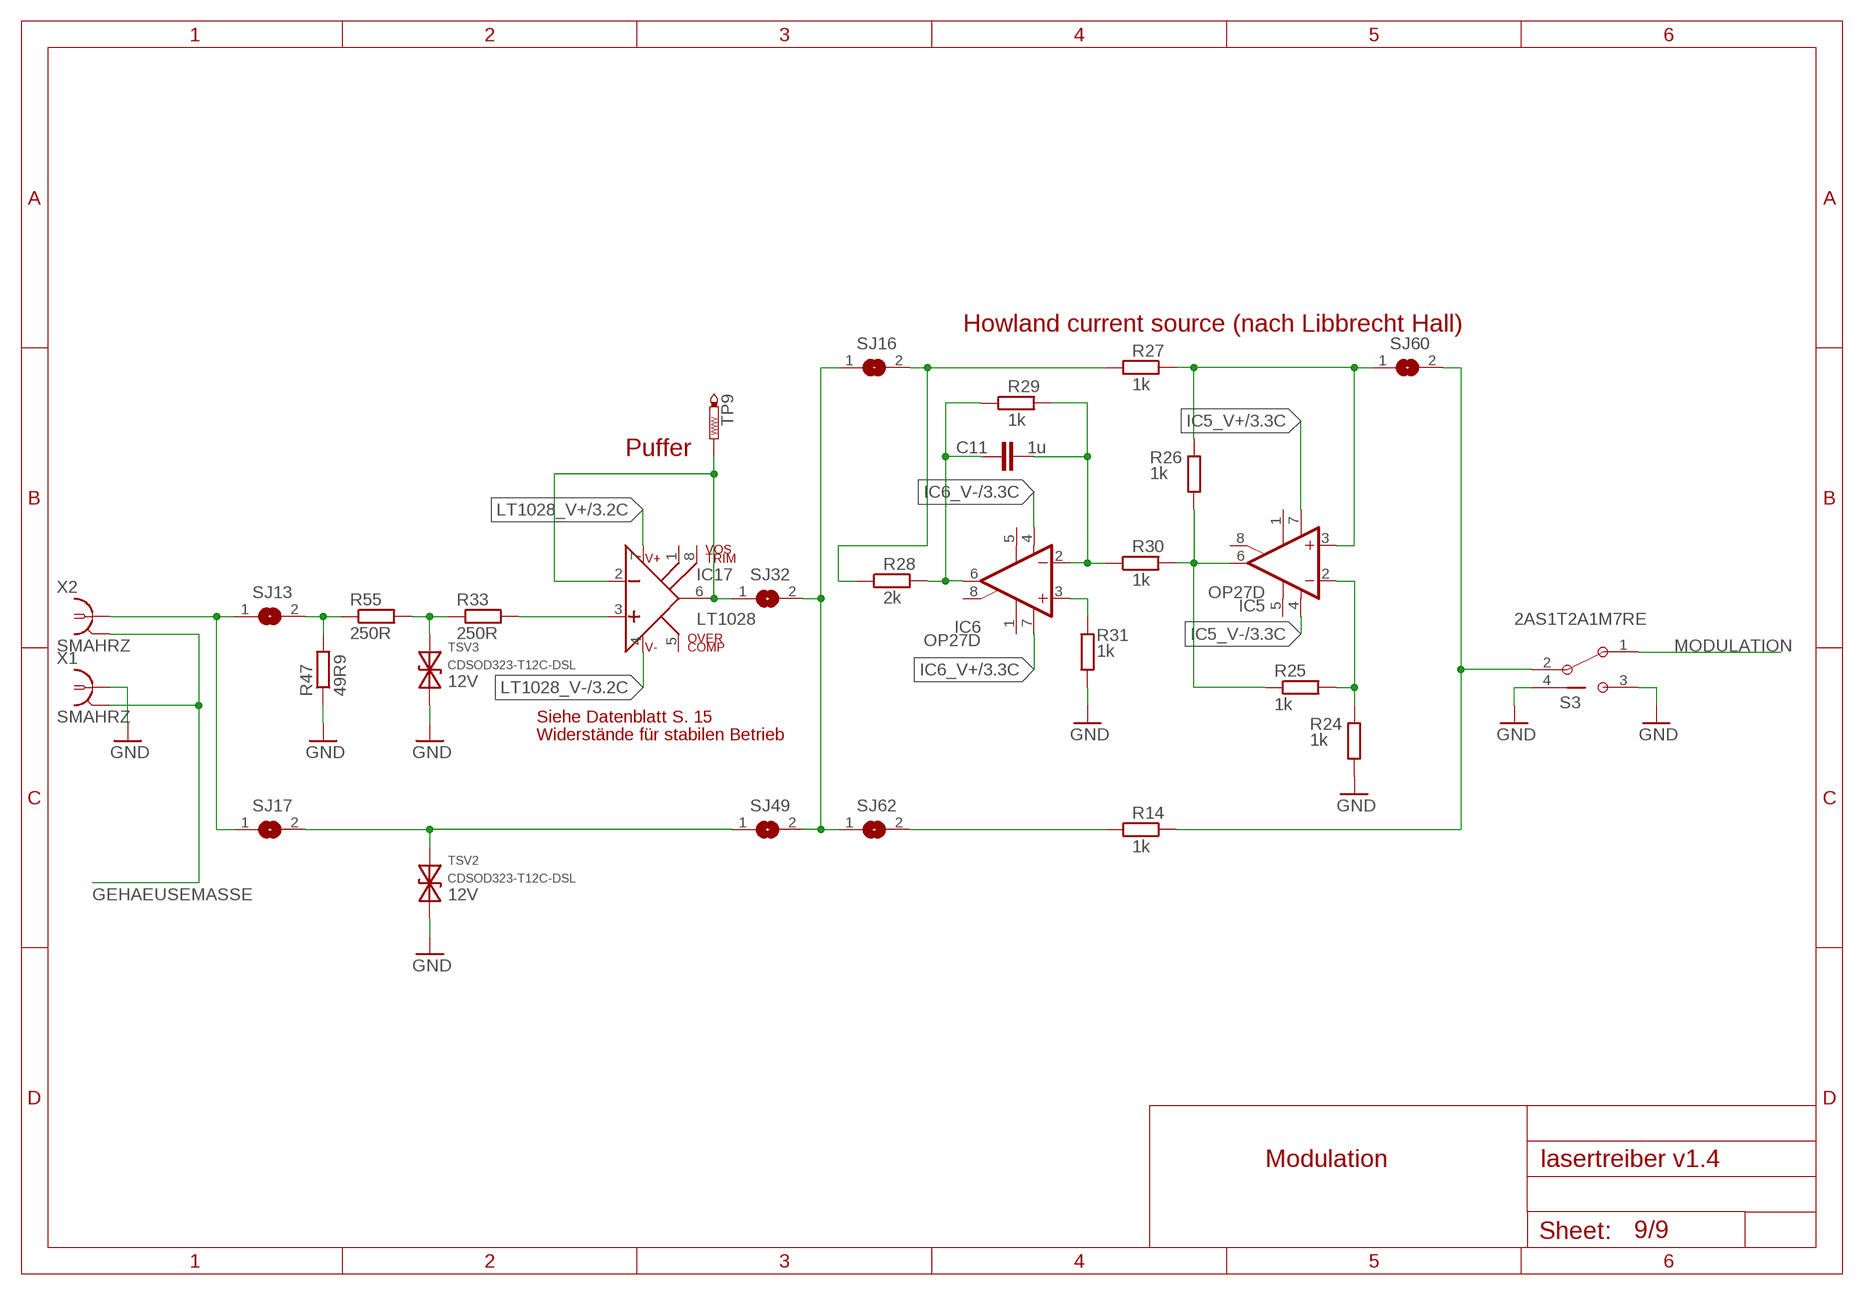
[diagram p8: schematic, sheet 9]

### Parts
C11  1u  C50X75  [C050-050X075]
IC5  OP27D  [SO08]
IC6  OP27D  [SO08]
IC17  LT1028  [SOIC8]
R14  1k  R1206  [R1206]
R24  1k  R0805  [R0805]
R25  1k  R0805  [R0805]
R26  1k  R0805  [R0805]
R27  1k  R1206  [R1206]
R28  2k  R0805  [R0805]
R29  1k  R0805  [R0805]
R30  1k  R0805  [R0805]
R31  1k  R0805  [R0805]
R33  250R  R0805  [R0805]
R47  49R9  R0805  [R0805]
R55  250R  R0805  [R0805]
S3  2AS1T2A1M7RE  [2AS1T2A1M7RE]
SJ13  SJ  [SJ]
SJ16  SJ  [SJ]
SJ17  SJ  [SJ]
SJ32  SJ  [SJ]
SJ49  SJ  [SJ]
SJ60  SJ  [SJ]
SJ62  SJ  [SJ]
TP9  PTR1PAD1-13  [P1-13]
TSV2  CDSOD323-T12C-DSL  CDSOD323-TXXSC''  [SOD323-W]
TSV3  CDSOD323-T12C-DSL  CDSOD323-TXXSC''  [SOD323-W]
X1  SMAHRZ  [SMA20_HRZ]
X2  SMAHRZ  [SMA20_HRZ]

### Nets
GEHAEUSEMASSE: X1.GND@1 X1.GND@2 X1.GND@3 X1.GND@4 X2.GND@1 X2.GND@2 X2.GND@3 X2.GND@4 ; also sheet 7
GND: R24.2 R31.2 R47.1 S3.3(A2) S3.4(GND) TSV2.C TSV3.C X1.SIGNAL ; also sheet 2,3,4,5,6,7,8
IC5_V+: IC5.7(V+) ; also sheet 3
IC5_V-: IC5.4(V-) ; also sheet 3
IC6_V+: IC6.7(V+) ; also sheet 3
IC6_V-: IC6.4(V-) ; also sheet 3
LT1028_V+: IC17.7(+VS) ; also sheet 3
LT1028_V-: IC17.4(-VS) ; also sheet 3
MODULATION: S3.1(A1) ; also sheet 7
N$13: R14.2 SJ62.2
N$20: IC17.2(IN-) IC17.6(OUT) SJ32.1 TP9.TP
N$21: R33.1 R55.2 TSV3.A
N$23: SJ17.2 SJ49.1 TSV2.A
N$34: IC5.2(-IN) R24.1 R25.2
N$35: IC5.6(OUT) R25.1 R26.1 R30.2
N$36: C11.2 IC6.6(OUT) R28.2 R29.1
N$38: IC6.3(+IN) R31.1
N$39: C11.1 IC6.2(-IN) R29.2 R30.1
N$41: R14.1 S3.2(A) SJ60.2
N$42: IC5.3(+IN) R26.2 R27.1 SJ60.1
N$43: SJ16.1 SJ32.2 SJ49.2 SJ62.1
N$52: IC17.3(IN+) R33.2
N$65: R27.2 R28.1 SJ16.2
N$103: R47.2 R55.1 SJ13.2
N$111: SJ13.1 SJ17.1 X2.SIGNAL
Unconnected: IC5.1(ON1) IC5.5(OPT) IC5.8(ON2) IC6.1(ON1) IC6.5(OPT) IC6.8(ON2) IC17.1(VOSTRIM) IC17.5(OVERCOMP) IC17.8(VOSTRIM)

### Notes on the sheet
- Howland current source (nach Libbrecht Hall)
- Puffer
- 12V
- Siehe Datenblatt S. 15
- Widerstände für stabilen Betrieb
- 12V
- Modulation

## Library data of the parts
BOLZEN1-BOLZEN14 = lasertreiber:BOLZEN
BOX1-BOX3 = lasertreiber:BOX
C1 C8 C10-C13 C19 C23 C25 C27 C28 C31 C33-C35 C38 C41-C44 C49 C51 C54 C55 C57 C59 C61-C65 C69 C70 C74 = lasertreiber:C: Keramik- und Folienkondesatoren für Lasertreiber
C2-C7 C9 C14-C18 C24 C26 C29 C30 C32 C36 C37 C39 C40 C46-C48 C50 C52 C53 C56 C58 C60 C66 C68 C71-C73 = lasertreiber:C-POL: Polare Kondensatoren für den Lasertreiber
D1 D2 D5 D16 D17 = lasertreiber:DIODE: Dioden für Lasertreiber
D3 = lasertreiber:BZX84
GEHAEUSE1 = lasertreiber:GEHAEUSEMASSE
IC1 IC4 = lasertreiber:LM317
IC2 = linear:LM399H: Precision Z DIODE
IC3 = lasertreiber:LT3045
IC5 IC6 = linear:OP27: OP AMP
IC10 = lasertreiber:LT1236: Integrierte Schaltkreise
IC14 IC16 = lasertreiber:AD8429: AD8429 Datasheet
IC17 = lasertreiber:LT1028: LT1028 Datasheet
JP1 = lasertreiber:IL-G
L1-L8 L11-L24 = lasertreiber:L
LASORB1 = lasertreiber:LASORB
LED1-LED3 = lasertreiber:LED: LED
Q2 = lasertreiber:BCP
Q3 = lasertreiber:IRF512: N-CHANNEL MOS FET
R1-R5 R8-R19 R21-R37 R39 R41-R59 R62-R68 = lasertreiber:R
R6 R7 R20 R38 R40 R60 R61 = lasertreiber:POTENTIOMETER_: Potentiometer
S1 = lasertreiber:1MD1T2B4M7QE
S2 S3 = lasertreiber:2AS1T2A1M7RE
SJ1-SJ51 SJ56 SJ57 SJ60 SJ62 = jumper:SJ: SMD solder JUMPER
ST1 = Ringdown Rev 2.01:A.KO-09_MAC64LE: 64 poliger A/C Steckverbinder für 19" Einschub
T1 T2 = lasertreiber:BC857C: PNP Epitaxial Silicon Transistor
T3 = lasertreiber:IRLML9301: MOS FET
T4 = lasertreiber:IRLML0060
TP1-TP11 = testpad:PTR1: TEST PIN
TSV1-TSV3 = lasertreiber:CDSOD323-TXXSC
U1 = lasertreiber:LTC6655
X1 X2 X6 X7 = lasertreiber:SMA
X3 = lasertreiber:PINHEADER-8
X4 = lasertreiber:PINHEADER-10
X5 = con-thomas-betts:D-SUB9-: D-Subminiatur Connector Source: Electronioc Interconnects European Edition 1998; OC_FARNELL: unknown; OC_NEWARK: unknown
